| IBIS file rt600_114wlcsp_dr2.ibs generated by Viper version: 2020.06.10
[IBIS Ver]   5.0
[Comment Char]   |_char
[File Name]   rt600_114wlcsp_dr2.ibs
[File Rev]   1.3
[Date]   Wed Jun 10 15:09:24 2020
[Source]   NXP Viper 2020.06.10
[Notes]
[Disclaimer] IMPORTANT NOTICE
  This information is provided on an AS IS basis and without warranty.
  IN NO EVENT SHALL NXP BE LIABLE FOR INCIDENTAL OR CONSEQUENTIAL
  DAMAGES ARISING FROM USE OF THIS INFORMATION. THIS DISCLAIMER OF
  WARRANTY EXTENDS TO THE USER OF THE INFORMATION, AND TO THEIR CUSTOMERS
  OR USERS OF PRODUCTS  AND IS IN LIEU OF ALL WARRANTIES WHETHER EXPRESS,
  IMPLIED, OR STATUTORY, INCLUDING IMPLIED WARRANTIES OF MERCHANTABILITY
  OR FITNESS FOR PARTICULAR PURPOSE.
  NXP does not represent or warrant that the information furnished
  hereunder is free of infringement of any third party patents,
  copyrights, trade secrets, or other intellectual property rights.
  NXP does not represent or warrant that the information is free of
  defect, or that it meets any particular standard, requirements or need
  of the user of the infomation or their customers.
  NXP reserves the right to change the information in this file
  without notice.
   http://www.nxp.com
[Copyright]   (C) Copyright NXP 2004 - 2020, All Rights Reserved.
|   114WLCSP
[Component]   114WLCSP
[Manufacturer]   NXP
[Package]
| variable   typ   min   max
R_pkg   0.24438   0.016619   0.63766
L_pkg   5.140e-10   1.147e-10   1.162e-09
C_pkg   2.651e-13   1.722e-13   4.529e-13
[Pin] signal_name   model_name   R_pin   L_pin   C_pin
A1   GND   GND   NA   NA   NA
A2   PIO2_19   gpio   0.20048   4.395e-10 2.429e-13
A3   PIO2_21   gpio   0.28201   5.946e-10 2.735e-13
A5   PIO1_23   sd_mmc   0.050875  2.154e-10 2.090e-13
A6   GND   GND   NA   NA   NA
A7   PIO3_27   gpio   0.022239  1.242e-10 1.916e-13
A8   PIO3_26   gpio   0.19523   4.219e-10 2.405e-13
A9   VDD1V8   POWER   NA   NA   NA
A10   VDDCORE   POWER   NA   NA   NA
A11   GND   GND   NA   NA   NA
B1   PIO2_18   gpio   0.022426  1.268e-10 1.845e-13
B2   PIO1_17   gpio   0.16691   3.734e-10 2.300e-13
B3   PIO2_16   gpio   0.31823   6.366e-10 2.844e-13
B4   PIO1_19   sd_mmc   0.20453   4.621e-10 2.429e-13
B5   PIO1_22   sd_mmc   0.21837   4.602e-10 2.459e-13
B6   GND   GND   NA   NA   NA
B7   PIO1_18   sd_mmc   0.24821   5.078e-10 2.594e-13
B8   VDDE0   POWER   NA   NA   NA
B9   USB0_DM   NC   0.18639   4.495e-10 2.705e-13
B10   USB0_DP   NC   0.202   4.723e-10 2.783e-13
C1   VDDCORE   POWER   NA   NA   NA
C2   PIO1_15   gpio   0.16403   3.597e-10 2.285e-13
C3   PIO1_16   gpio   0.30454   6.201e-10 2.821e-13
C4   PIO2_17   gpio   0.46815   8.989e-10 3.425e-13
C5   PIO2_20   gpio   0.59303   1.103e-09 3.884e-13
C6   PIO1_20   sd_mmc   0.40745   7.830e-10 3.199e-13
C7   PIO1_21   sd_mmc   0.49032   9.113e-10 3.439e-13
C8   PIO2_28   gpio   0.34787   6.788e-10 2.979e-13
C9   PIO2_30   gpio   0.24948   5.092e-10 2.615e-13
C10   VDD_USB33   POWER   NA   NA   NA
C11   PIO2_29   gpio   0.034744  1.762e-10 1.953e-13
D2   PIO1_12   gpio   0.16593   3.667e-10 2.249e-13
D3   PIO1_13   gpio   0.27011   5.631e-10 2.690e-13
D4   PIO1_14   gpio   0.3802   7.385e-10 3.071e-13
D5   VDD18_IOREF   POWER   NA   NA   NA
D6   GND   GND   NA   NA   NA
D7   VDDE0   POWER   NA   NA   NA
D8   PIO2_25   gpio   0.35751   6.876e-10 3.006e-13
D9   PIO2_27   gpio   0.24624   5.053e-10 2.592e-13
D10   PIO2_26   gpio   0.14024   3.325e-10 2.195e-13
E1   PIO0_11   gpio   0.030779  1.565e-10 1.943e-13
E2   PIO0_10   gpio   0.16758   3.654e-10 2.258e-13
E3   PIO0_9   gpio   0.25715   5.360e-10 2.654e-13
E4   PIO0_8   gpio   0.36068   7.123e-10 3.029e-13
E5   PIO1_11   gpio   0.4749   8.605e-10 3.550e-13
E6   GND   GND   NA   NA   NA
E7   VDDE0   POWER   NA   NA   NA
E8   VDDCORE   POWER   NA   NA   NA
E9   VDDE1   POWER   NA   NA   NA
E10   PIO1_10   gpio   0.15965   3.531e-10 2.231e-13
E11   PIO1_5   gpio   0.025492  1.567e-10 1.880e-13
F1   VDDCORE   POWER   NA   NA   NA
F2   VDDE0   POWER   NA   NA   NA
F3   PIO0_7   gpio   0.27314   5.437e-10 2.667e-13
F4   PIO0_3   gpio   0.39471   7.653e-10 3.135e-13
F5   PIO0_2   gpio   0.50641   9.330e-10 3.496e-13
F6   VDDCORE   POWER   NA   NA   NA
F7   VDDCORE   POWER   NA   NA   NA
F8   GND   GND   NA   NA   NA
F9   PIO1_4   gpio   0.25086   5.021e-10 2.613e-13
F10   PIO1_3   gpio   0.15449   3.389e-10 2.269e-13
F11   GND   GND   NA   NA   NA
G1   PIO0_4   gpio   0.022136  1.327e-10 1.857e-13
G2   VDDCORE   POWER   NA   NA   NA
G3   VDDE0   POWER   NA   NA   NA
G4   PIO0_13   gpio   0.42065   7.978e-10 3.215e-13
G5   PIO2_14   gpio   0.63766   1.162e-09 4.142e-13
G6   GND   GND   NA   NA   NA
G7   VDDCORE   POWER   NA   NA   NA
G8   VDD_PLL18   POWER   NA   NA   NA
G9   VDD_FUSE18   POWER   NA   NA   NA
G10   VDDCORE   POWER   NA   NA   NA
G11   VDDCORE   POWER   NA   NA   NA
H2   PIO0_1   gpio   0.15642   3.455e-10 2.200e-13
H3   PIO0_0   gpio   0.24376   5.083e-10 2.587e-13
H4   PIO2_15   gpio   0.4777   8.957e-10 3.542e-13
H5   PIO0_20   gpio   0.44654   8.564e-10 3.349e-13
H6   PIO0_19   gpio   0.51584   9.626e-10 3.593e-13
H7   PIO0_22   gpio   0.47175   8.818e-10 3.430e-13
H8   PIO0_24   gpio   0.49283   9.192e-10 3.514e-13
H9   LDO_ENABLE   gpio   0.20869   6.650e-10 4.529e-13
H10   VDD1V8_DRV   POWER   NA   NA   NA
H11   VDD18_IOREF   POWER   NA   NA   NA
J1   PIO0_6   gpio   0.0173   1.277e-10 1.723e-13
J2   VDDE0   POWER   NA   NA   NA
J3   PIO0_5   gpio   0.24173   4.937e-10 2.531e-13
J4   PIO0_27   gpio   0.29885   6.122e-10 2.806e-13
J5   PIO1_8   gpio   0.27596   5.771e-10 2.486e-13
J6   PIO0_15   gpio   0.37062   7.317e-10 3.058e-13
J7   PIO2_31   gpio   0.37085   7.257e-10 3.064e-13
J8   VDDE1   POWER   NA   NA   NA
J9   GND   GND   NA   NA   NA
J10   VDD1V8_DRV   POWER   NA   NA   NA
J11   GND   GND   NA   NA   NA
K1   PIO0_12   gpio   0.019028  1.147e-10 1.768e-13
K2   VDD1V8   POWER   NA   NA   NA
K3   PIO1_9   gpio   0.19002   4.108e-10 2.400e-13
K4   PIO0_14   gpio   0.18013   4.160e-10 2.354e-13
K5   PIO0_16   gpio   0.19208   4.404e-10 2.406e-13
K6   PIO1_2   gpio   0.2013   4.476e-10 2.425e-13
K7   PIO0_23   gpio   0.24072   5.038e-10 2.560e-13
K8   PIO0_29   gpio   0.23731   4.830e-10 2.505e-13
K9   XTALINSYS   NC   0.10247   2.885e-10 2.173e-13
K10   RESETN   gpio   0.10678   3.488e-10 2.858e-13
L1   GND   GND   NA   NA   NA
L2   VDDE1   POWER   NA   NA   NA
L3   PIO0_26   gpio   0.016734  1.276e-10 1.751e-13
L5   PIO0_21   gpio   0.028366  1.844e-10 1.897e-13
L6   PIO0_25   gpio   0.035236  1.818e-10 1.955e-13
L7   GND   GND   NA   NA   NA
L8   PIO0_30   gpio   0.12146   2.973e-10 2.125e-13
L9   XTALOUTSYS   NC   0.016619  1.147e-10 1.722e-13
L10   VDD1V8   POWER   NA   NA   NA
L11   VDD_AO18   POWER   NA   NA   NA
[Pin Mapping]   pulldown_ref   pullup_ref
A1   GND   NC
A2   GND   VDDE0
A3   GND   VDDE0
A5   GND   VDDE0
A6   GND   NC
A7   GND   VDDE0
A8   GND   VDDE0
A9   NC   VDD1V8
A10   NC   VDDCORE
A11   GND   NC
B1   GND   VDDE0
B2   GND   VDDE0
B3   GND   VDDE0
B4   GND   VDDE0
B5   GND   VDDE0
B6   GND   NC
B7   GND   VDDE0
B8   NC   VDDE0
B9   NC   NC
B10   NC   NC
C1   NC   VDDCORE
C2   GND   VDDE0
C3   GND   VDDE0
C4   GND   VDDE0
C5   GND   VDDE0
C6   GND   VDDE0
C7   GND   VDDE0
C8   GND   VDDE1
C9   GND   VDDE1
C10   NC   VDD_USB33
C11   GND   VDDE1
D2   GND   VDDE0
D3   GND   VDDE0
D4   GND   VDDE0
D5   NC   VDD18_IOREF
D6   GND   NC
D7   NC   VDDE0
D8   GND   VDDE1
D9   GND   VDDE1
D10   GND   VDDE1
E1   GND   VDDE0
E2   GND   VDDE0
E3   GND   VDDE0
E4   GND   VDDE0
E5   GND   VDDE0
E6   GND   NC
E7   NC   VDDE0
E8   NC   VDDCORE
E9   NC   VDDE1
E10   GND   VDDE1
E11   GND   VDDE1
F1   NC   VDDCORE
F2   NC   VDDE0
F3   GND   VDDE0
F4   GND   VDDE0
F5   GND   VDDE0
F6   NC   VDDCORE
F7   NC   VDDCORE
F8   GND   NC
F9   GND   VDDE1
F10   GND   VDDE1
F11   GND   NC
G1   GND   VDDE0
G2   NC   VDDCORE
G3   NC   VDDE0
G4   GND   VDDE0
G5   GND   VDDE0
G6   GND   NC
G7   NC   VDDCORE
G8   NC   VDD_PLL18
G9   NC   VDD_FUSE18
G10   NC   VDDCORE
G11   NC   VDDCORE
H2   GND   VDDE0
H3   GND   VDDE0
H4   GND   VDDE0
H5   GND   VDDE1
H6   GND   VDDE1
H7   GND   VDDE1
H8   GND   VDDE1
H9   GND   VDD_AO18
H10   NC   VDD1V8_DRV
H11   NC   VDD18_IOREF
J1   GND   VDDE0
J2   NC   VDDE0
J3   GND   VDDE0
J4   GND   VDDE1
J5   GND   VDDE1
J6   GND   VDDE1
J7   GND   VDDE1
J8   NC   VDDE1
J9   GND   NC
J10   NC   VDD1V8_DRV
J11   GND   NC
K1   GND   VDDE0
K2   NC   VDD1V8
K3   GND   VDDE1
K4   GND   VDDE1
K5   GND   VDDE1
K6   GND   VDDE1
K7   GND   VDDE1
K8   GND   VDDE1
K9   NC   NC
K10   GND   VDD_AO18
L1   GND   NC
L2   NC   VDDE1
L3   GND   VDDE1
L5   GND   VDDE1
L6   GND   VDDE1
L7   GND   NC
L8   GND   VDDE1
L9   NC   NC
L10   NC   VDD1V8
L11   NC   VDD_AO18
|*   Model Selector   *
[Model Selector] gpio
io_obe1dse0sre0   5mA current driving capability, without slew rate
io_obe1dse0sre1   5mA current driving capability, with slew rate
io_obe1dse1sre0   10mA current driving capability, without slew rate
io_obe1dse1sre1   10mA current driving capability, with slew rate
[Model Selector] sd_mmc
BDPROGSCARUDQP_SDMMC_3V3SF_00_SD   PSW=0 PDRV=0 MODE=1V8 SD
BDPROGSCARUDQP_SDMMC_3V3SF_01_SD   PSW=0 PDRV=1 MODE=1V8 SD
BDPROGSCARUDQP_SDMMC_3V3SF_00_MMC   PSW=0 PDRV=0 MODE=1V8 MMC
BDPROGSCARUDQP_SDMMC_3V3SF_01_MMC   PSW=0 PDRV=1 MODE=1V8 MMC
BDPROGSCARUDQP_SDMMC_3V3SF_10   PSW=1 PDRV=0 MODE=3V3 SD & 3V3 MMC
BDPROGSCARUDQP_SDMMC_3V3SF_11   PSW=1 PDRV=1 MODE=3V3 SD & 3V3 MMC
BDPROGSCARUDQP_SDMMC_3V3SF_11_2v7   PSW=1 PDRV=1 MODE=2V7 SD & 2V7 MMC
BDPROGSCARUDQP_SDMMC_3V3SF_10_2v7   PSW=1 PDRV=0 MODE=2V7 SD & 2V7 MMC
| End [Component] 114WLCSP
| Models and submodels in the file (12): BDPROGSCARUDQP_SDMMC_3V3SF_00_MMC (I/O), BDPROGSCARUDQP_SDMMC_3V3SF_00_SD (I/O), BDPROGSCARUDQP_SDMMC_3V3SF_01_MMC (I/O), BDPROGSCARUDQP_SDMMC_3V3SF_01_SD (I/O), BDPROGSCARUDQP_SDMMC_3V3SF_10 (I/O), BDPROGSCARUDQP_SDMMC_3V3SF_10_2v7 (I/O), BDPROGSCARUDQP_SDMMC_3V3SF_11 (I/O), BDPROGSCARUDQP_SDMMC_3V3SF_11_2v7 (I/O), io_obe1dse0sre0 (I/O), io_obe1dse0sre1 (I/O), io_obe1dse1sre0 (I/O), io_obe1dse1sre1 (I/O)
